DATA_BLOCK "DB_Gest_ES"
TITLE =
{ S7_language := '9(1) Angielski (Stany Zjednoczone)  11.01.2022  09:45:15' }
VERSION : 0.1


  STRUCT
   CMD : STRUCT
    StartVentilazione_Zona1 : BOOL ;	//Zona 1 +31FAN01
    StartVentilazione_Zona2 : BOOL ;	//Zona 2 +71FAN01
    SPARE_CMD0_02 : BOOL ;
    SPARE_CMD0_03 : BOOL ;
    StopVentilazione_Zona1 : BOOL ;
    StopVentilazione_Zona2 : BOOL ;
    VentilazioneRid_Zona1 : BOOL ;	//Ventilazione Ridotta Zona1
    VentilazioneRid_Zona2 : BOOL ;	//Ventilazione Ridotta Zona2
    Start_Riscarldo_Forno1 : BOOL ;
    Start_Riscarldo_Forno2 : BOOL ;
    AssenzaScoccheCabina : BOOL ;	//Assenza scocche cabina smalto
    SPARE_CMD1_03 : BOOL ;
    Stop_Riscarldo_Forno1 : BOOL ;
    Stop_Riscarldo_Forno2 : BOOL ;
    SPARE_CMD1_06 : BOOL ;
    SPARE_CMD1_07 : BOOL ;
    SPARE_CMD2_00 : BOOL ;
    SPARE_CMD2_01 : BOOL ;
    Forno2_PE_In_CMD2_02 : BOOL ;	//Scocca in ingresso Forno 2
    SPARE_CMD2_03 : BOOL ;
    SPARE_CMD2_04 : BOOL ;
    SPARE_CMD2_05 : BOOL ;
    SPARE_CMD2_06 : BOOL ;
    SPARE_CMD2_07 : BOOL ;
    SPARE_CMD3_00 : BOOL ;
    SPARE_CMD3_01 : BOOL ;
    SPARE_CMD3_02 : BOOL ;
    SPARE_CMD3_03 : BOOL ;
    SPARE_CMD3_04 : BOOL ;
    SPARE_CMD3_05 : BOOL ;
    SPARE_CMD3_06 : BOOL ;
    SPARE_CMD3_07 : BOOL ;
   END_STRUCT ;
   STS : STRUCT
    SPARE_STS0_00 : BOOL ;
    SPARE_STS0_01 : BOOL ;
    SPARE_STS0_02 : BOOL ;
    SPARE_STS0_03 : BOOL ;
    SPARE_STS0_04 : BOOL ;
    SPARE_STS0_05 : BOOL ;
    SPARE_STS0_06 : BOOL ;
    SPARE_STS0_07 : BOOL ;
    SPARE_STS1_00 : BOOL ;
    SPARE_STS1_01 : BOOL ;
    SPARE_STS1_02 : BOOL ;
    SPARE_STS1_03 : BOOL ;
    SPARE_STS1_04 : BOOL ;
    SPARE_STS1_05 : BOOL ;
    SPARE_STS1_06 : BOOL ;
    SPARE_STS1_07 : BOOL ;
    SPARE_STS2_00 : BOOL ;
    SPARE_STS2_01 : BOOL ;
    SPARE_STS2_02 : BOOL ;
    SPARE_STS2_03 : BOOL ;
    SPARE_STS2_04 : BOOL ;
    SPARE_STS2_05 : BOOL ;
    SPARE_STS2_06 : BOOL ;
    SPARE_STS2_07 : BOOL ;
    SPARE_STS3_00 : BOOL ;
    SPARE_STS3_01 : BOOL ;
    SPARE_STS3_02 : BOOL ;
    SPARE_STS3_03 : BOOL ;
    SPARE_STS3_04 : BOOL ;
    SPARE_STS3_05 : BOOL ;
    SPARE_STS3_06 : BOOL ;
    SPARE_STS3_07 : BOOL ;
   END_STRUCT ;
   Cnt_9PU1 : INT ;
   Cnt_8PU1 : INT ;
   Cnt_9RC : INT ;
   Cnt_8RC : INT ;
   Soglie : ARRAY  [1 .. 20 ] OF INT ;
   SetPoint : ARRAY  [1 .. 20 ] OF INT ;
   SPARE : ARRAY  [1 .. 20 ] OF INT ;
   FLAG : STRUCT
    _000 : BOOL ;	//Abilita Gestione Risparmio Energetico
    _001 : BOOL ;	//Stop Raffreddamento Linea 1
    _002 : BOOL ;	//Stop Raffreddamento Linea 2
    _003 : BOOL ;	//Stop Riscaldamento Linea 1
    _004 : BOOL ;	//Stop Riscaldamento Linea 2
    _005 : BOOL ;	//Forno 2 spento da Calendario
    _006 : BOOL ;	//RESERVE
    _007 : BOOL ;	//RESERVE
    _008 : BOOL ;	//RESERVE
    _009 : BOOL ;	//RESERVE
    _010 : BOOL ;	//RESERVE
    _011 : BOOL ;	//START COOLING ZONE Linea 1
    _012 : BOOL ;	//START COOLING ZONE Linea 2
    _013 : BOOL ;	//Start Raffreddamento Linea 1
    _014 : BOOL ;	//Start Raffreddamento Linea 2
    _015 : BOOL ;	//RESERVE
    _016 : BOOL ;	//RESERVE
    _017 : BOOL ;	//RESERVE
    _018 : BOOL ;	//RESERVE
    _019 : BOOL ;	//RESERVE
    _020 : BOOL ;	//RESERVE
    _021 : BOOL ;	//Riduzione Frequenza Raffreddamento Linea 1
    _022 : BOOL ;	//Riduzione Frequenza Raffreddamento Linea 2
    _023 : BOOL ;	//RESERVE
    _024 : BOOL ;	//RESERVE
    _025 : BOOL ;	//RESERVE
    _026 : BOOL ;	//RESERVE
    _027 : BOOL ;	//RESERVE
    _028 : BOOL ;	//RESERVE
    _029 : BOOL ;	//RESERVE
    _030 : BOOL ;	//AUX CONSENSO ACCENZIONE PRIMER
    _031 : BOOL ;	//ONS COMANDO ACCENSIONE PRIMER
    _032 : BOOL ;	//CMD STOP PRIMER
    _033 : BOOL ;	//Comando Accensione Manuale
    _034 : BOOL ;	//RESERVE
    _035 : BOOL ;	//RESERVE
    _036 : BOOL ;	//RESERVE
    _037 : BOOL ;	//RESERVE
    _038 : BOOL ;	//RESERVE
    _039 : BOOL ;	//AUX CONSENSO ACCENZIONE FORNO 2
    _040 : BOOL ;	//AUX CONSENSO ACCENZIONE FORNO 1
    _041 : BOOL ;	//ONS COMANDO ACCENSIONE FORNO 2
    _042 : BOOL ;	//ONS COMANDO ACCENSIONE FORNO 1
    _043 : BOOL ;	//RESERVE
    _044 : BOOL ;	//RESERVE
    _045 : BOOL ;	//RESERVE
    _046 : BOOL ;	//RESERVE
    _047 : BOOL ;	//RESERVE
    _048 : BOOL ;	//RESERVE
    _049 : BOOL ;	//RESERVE
    _050 : BOOL ;	//Ons Comando OFF senza calendario
    _051 : BOOL ;	//RESERVE
    _052 : BOOL ;	//RESERVE
    _053 : BOOL ;	//RESERVE
    _054 : BOOL ;	//RESERVE
    _055 : BOOL ;	//RESERVE
    _056 : BOOL ;	//RESERVE
    _057 : BOOL ;	//RESERVE
    _058 : BOOL ;	//RESERVE
    _059 : BOOL ;	//RESERVE
    _060 : BOOL ;	//RESERVE
    _061 : BOOL ;	//RESERVE
    _062 : BOOL ;	//RESERVE
    _063 : BOOL ;	//RESERVE
    _064 : BOOL ;	//RESERVE
    _065 : BOOL ;	//RESERVE
    _066 : BOOL ;	//RESERVE
    _067 : BOOL ;	//RESERVE
    _068 : BOOL ;	//RESERVE
    _069 : BOOL ;	//Abilita Gestione Risparmio Energetico FLA
    _070 : BOOL ;	//Start 43FLA02
    _071 : BOOL ;	//Start 44FLA02
    _072 : BOOL ;	//Start 51FLA02
    _073 : BOOL ;	//Start 52FLA02
    _074 : BOOL ;	//RESERVE
    _075 : BOOL ;	//RESERVE
    _076 : BOOL ;	//RESERVE
    _077 : BOOL ;	//Estate
    _078 : BOOL ;	//Temperato
    _079 : BOOL ;	//Inverno
    _080 : BOOL ;	//Modalita 1 Estate
    _081 : BOOL ;	//Modalita 1 Inverno
    _082 : BOOL ;	//Stop gruppo 84PP31-M1
    _083 : BOOL ;	//RESERVE
    _084 : BOOL ;	//RESERVE
    _085 : BOOL ;	//RESERVE
    _086 : BOOL ;	//RESERVE
    _087 : BOOL ;	//RESERVE
    _088 : BOOL ;	//RESERVE
    _089 : BOOL ;	//RESERVE
    _090 : BOOL ;	//RESERVE
    _091 : BOOL ;	//RESERVE
    _092 : BOOL ;	//RESERVE
    _093 : BOOL ;	//RESERVE
    _094 : BOOL ;	//RESERVE
    _095 : BOOL ;	//RESERVE
    _096 : BOOL ;	//RESERVE
    _097 : BOOL ;	//RESERVE
    _098 : BOOL ;	//RESERVE
    _099 : BOOL ;	//RESERVE
    _100 : BOOL ;	//RESERVE
   END_STRUCT ;
   ONS : ARRAY  [1 .. 20 ] OF BOOL ;
   Tmr : STRUCT
    Delay_01 : INT ;	//TMR Delay
    ONS_Delay_01 : BOOL ;	//Ons TMR Delay
    EN_Delay_01 : BOOL ;	//En TMR Delay
    DN_Delay_01 : BOOL ;	//DN TMR Delay
    Delay_02 : INT ;	//TMR Delay
    ONS_Delay_02 : BOOL ;	//Ons TMR Delay
    EN_Delay_02 : BOOL ;	//En TMR Delay
    DN_Delay_02 : BOOL ;	//DN TMR Delay
    Delay_03 : INT ;	//TMR Delay
    ONS_Delay_03 : BOOL ;	//Ons TMR Delay
    EN_Delay_03 : BOOL ;	//En TMR Delay
    DN_Delay_03 : BOOL ;	//DN TMR Delay
    Delay_04 : INT ;	//TMR Delay
    ONS_Delay_04 : BOOL ;	//Ons TMR Delay
    EN_Delay_04 : BOOL ;	//En TMR Delay
    DN_Delay_04 : BOOL ;	//DN TMR Delay
    Delay_05 : INT ;	//TMR Delay
    ONS_Delay_05 : BOOL ;	//Ons TMR Delay
    EN_Delay_05 : BOOL ;	//En TMR Delay
    DN_Delay_05 : BOOL ;	//DN TMR Delay
    Delay_06 : INT ;	//TMR Delay
    ONS_Delay_06 : BOOL ;	//Ons TMR Delay
    EN_Delay_06 : BOOL ;	//En TMR Delay
    DN_Delay_06 : BOOL ;	//DN TMR Delay
    Delay_07 : INT ;	//TMR Delay
    ONS_Delay_07 : BOOL ;	//Ons TMR Delay
    EN_Delay_07 : BOOL ;	//En TMR Delay
    DN_Delay_07 : BOOL ;	//DN TMR Delay
    Delay_08 : INT ;	//TMR Delay
    ONS_Delay_08 : BOOL ;	//Ons TMR Delay
    EN_Delay_08 : BOOL ;	//En TMR Delay
    DN_Delay_08 : BOOL ;	//DN TMR Delay
    Delay_09 : INT ;	//TMR Delay
    ONS_Delay_09 : BOOL ;	//Ons TMR Delay
    EN_Delay_09 : BOOL ;	//En TMR Delay
    DN_Delay_09 : BOOL ;	//DN TMR Delay
    Delay_10 : INT ;	//TMR Delay
    ONS_Delay_10 : BOOL ;	//Ons TMR Delay
    EN_Delay_10 : BOOL ;	//En TMR Delay
    DN_Delay_10 : BOOL ;	//DN TMR Delay
   END_STRUCT ;
  END_STRUCT ;
BEGIN
   CMD.StartVentilazione_Zona1 := FALSE;
   CMD.StartVentilazione_Zona2 := FALSE;
   CMD.SPARE_CMD0_02 := FALSE;
   CMD.SPARE_CMD0_03 := FALSE;
   CMD.StopVentilazione_Zona1 := TRUE;
   CMD.StopVentilazione_Zona2 := TRUE;
   CMD.VentilazioneRid_Zona1 := TRUE;
   CMD.VentilazioneRid_Zona2 := TRUE;
   CMD.Start_Riscarldo_Forno1 := FALSE;
   CMD.Start_Riscarldo_Forno2 := FALSE;
   CMD.AssenzaScoccheCabina := FALSE;
   CMD.SPARE_CMD1_03 := FALSE;
   CMD.Stop_Riscarldo_Forno1 := TRUE;
   CMD.Stop_Riscarldo_Forno2 := TRUE;
   CMD.SPARE_CMD1_06 := FALSE;
   CMD.SPARE_CMD1_07 := FALSE;
   CMD.SPARE_CMD2_00 := FALSE;
   CMD.SPARE_CMD2_01 := FALSE;
   CMD.Forno2_PE_In_CMD2_02 := FALSE;
   CMD.SPARE_CMD2_03 := FALSE;
   CMD.SPARE_CMD2_04 := FALSE;
   CMD.SPARE_CMD2_05 := FALSE;
   CMD.SPARE_CMD2_06 := FALSE;
   CMD.SPARE_CMD2_07 := FALSE;
   CMD.SPARE_CMD3_00 := FALSE;
   CMD.SPARE_CMD3_01 := FALSE;
   CMD.SPARE_CMD3_02 := FALSE;
   CMD.SPARE_CMD3_03 := FALSE;
   CMD.SPARE_CMD3_04 := FALSE;
   CMD.SPARE_CMD3_05 := FALSE;
   CMD.SPARE_CMD3_06 := FALSE;
   CMD.SPARE_CMD3_07 := FALSE;
   STS.SPARE_STS0_00 := FALSE;
   STS.SPARE_STS0_01 := FALSE;
   STS.SPARE_STS0_02 := FALSE;
   STS.SPARE_STS0_03 := FALSE;
   STS.SPARE_STS0_04 := FALSE;
   STS.SPARE_STS0_05 := FALSE;
   STS.SPARE_STS0_06 := FALSE;
   STS.SPARE_STS0_07 := FALSE;
   STS.SPARE_STS1_00 := FALSE;
   STS.SPARE_STS1_01 := FALSE;
   STS.SPARE_STS1_02 := FALSE;
   STS.SPARE_STS1_03 := FALSE;
   STS.SPARE_STS1_04 := FALSE;
   STS.SPARE_STS1_05 := FALSE;
   STS.SPARE_STS1_06 := FALSE;
   STS.SPARE_STS1_07 := FALSE;
   STS.SPARE_STS2_00 := FALSE;
   STS.SPARE_STS2_01 := FALSE;
   STS.SPARE_STS2_02 := FALSE;
   STS.SPARE_STS2_03 := FALSE;
   STS.SPARE_STS2_04 := FALSE;
   STS.SPARE_STS2_05 := FALSE;
   STS.SPARE_STS2_06 := FALSE;
   STS.SPARE_STS2_07 := FALSE;
   STS.SPARE_STS3_00 := FALSE;
   STS.SPARE_STS3_01 := FALSE;
   STS.SPARE_STS3_02 := FALSE;
   STS.SPARE_STS3_03 := FALSE;
   STS.SPARE_STS3_04 := FALSE;
   STS.SPARE_STS3_05 := FALSE;
   STS.SPARE_STS3_06 := FALSE;
   STS.SPARE_STS3_07 := FALSE;
   Cnt_9PU1 := 0;
   Cnt_8PU1 := 0;
   Cnt_9RC := 0;
   Cnt_8RC := 0;
   Soglie[1] := 0;
   Soglie[2] := 0;
   Soglie[3] := 0;
   Soglie[4] := 0;
   Soglie[5] := 0;
   Soglie[6] := 0;
   Soglie[7] := 0;
   Soglie[8] := 0;
   Soglie[9] := 0;
   Soglie[10] := 0;
   Soglie[11] := 0;
   Soglie[12] := 0;
   Soglie[13] := 0;
   Soglie[14] := 0;
   Soglie[15] := 0;
   Soglie[16] := 0;
   Soglie[17] := 0;
   Soglie[18] := 0;
   Soglie[19] := 0;
   Soglie[20] := 0;
   SetPoint[1] := 1800;
   SetPoint[2] := 1800;
   SetPoint[3] := 0;
   SetPoint[4] := 1500;
   SetPoint[5] := 60;
   SetPoint[6] := 60;
   SetPoint[7] := 100;
   SetPoint[8] := 200;
   SetPoint[9] := 3600;
   SetPoint[10] := 0;
   SetPoint[11] := 0;
   SetPoint[12] := 0;
   SetPoint[13] := 0;
   SetPoint[14] := 0;
   SetPoint[15] := 0;
   SetPoint[16] := 0;
   SetPoint[17] := 0;
   SetPoint[18] := 0;
   SetPoint[19] := 0;
   SetPoint[20] := 0;
   SPARE[1] := 0;
   SPARE[2] := 0;
   SPARE[3] := 0;
   SPARE[4] := 0;
   SPARE[5] := 0;
   SPARE[6] := 0;
   SPARE[7] := 0;
   SPARE[8] := 0;
   SPARE[9] := 0;
   SPARE[10] := 0;
   SPARE[11] := 0;
   SPARE[12] := 0;
   SPARE[13] := 0;
   SPARE[14] := 0;
   SPARE[15] := 0;
   SPARE[16] := 0;
   SPARE[17] := 0;
   SPARE[18] := 0;
   SPARE[19] := 0;
   SPARE[20] := 0;
   FLAG._000 := TRUE;
   FLAG._001 := FALSE;
   FLAG._002 := FALSE;
   FLAG._003 := FALSE;
   FLAG._004 := FALSE;
   FLAG._005 := FALSE;
   FLAG._006 := FALSE;
   FLAG._007 := FALSE;
   FLAG._008 := FALSE;
   FLAG._009 := FALSE;
   FLAG._010 := FALSE;
   FLAG._011 := FALSE;
   FLAG._012 := FALSE;
   FLAG._013 := TRUE;
   FLAG._014 := TRUE;
   FLAG._015 := FALSE;
   FLAG._016 := FALSE;
   FLAG._017 := FALSE;
   FLAG._018 := FALSE;
   FLAG._019 := FALSE;
   FLAG._020 := FALSE;
   FLAG._021 := FALSE;
   FLAG._022 := FALSE;
   FLAG._023 := FALSE;
   FLAG._024 := FALSE;
   FLAG._025 := FALSE;
   FLAG._026 := FALSE;
   FLAG._027 := FALSE;
   FLAG._028 := FALSE;
   FLAG._029 := FALSE;
   FLAG._030 := TRUE;
   FLAG._031 := FALSE;
   FLAG._032 := FALSE;
   FLAG._033 := FALSE;
   FLAG._034 := FALSE;
   FLAG._035 := FALSE;
   FLAG._036 := FALSE;
   FLAG._037 := FALSE;
   FLAG._038 := FALSE;
   FLAG._039 := TRUE;
   FLAG._040 := TRUE;
   FLAG._041 := FALSE;
   FLAG._042 := FALSE;
   FLAG._043 := FALSE;
   FLAG._044 := FALSE;
   FLAG._045 := FALSE;
   FLAG._046 := FALSE;
   FLAG._047 := FALSE;
   FLAG._048 := FALSE;
   FLAG._049 := FALSE;
   FLAG._050 := FALSE;
   FLAG._051 := FALSE;
   FLAG._052 := FALSE;
   FLAG._053 := FALSE;
   FLAG._054 := FALSE;
   FLAG._055 := FALSE;
   FLAG._056 := FALSE;
   FLAG._057 := FALSE;
   FLAG._058 := FALSE;
   FLAG._059 := FALSE;
   FLAG._060 := FALSE;
   FLAG._061 := FALSE;
   FLAG._062 := FALSE;
   FLAG._063 := FALSE;
   FLAG._064 := FALSE;
   FLAG._065 := FALSE;
   FLAG._066 := FALSE;
   FLAG._067 := FALSE;
   FLAG._068 := FALSE;
   FLAG._069 := FALSE;
   FLAG._070 := FALSE;
   FLAG._071 := FALSE;
   FLAG._072 := FALSE;
   FLAG._073 := FALSE;
   FLAG._074 := FALSE;
   FLAG._075 := FALSE;
   FLAG._076 := FALSE;
   FLAG._077 := FALSE;
   FLAG._078 := FALSE;
   FLAG._079 := FALSE;
   FLAG._080 := FALSE;
   FLAG._081 := FALSE;
   FLAG._082 := FALSE;
   FLAG._083 := FALSE;
   FLAG._084 := FALSE;
   FLAG._085 := FALSE;
   FLAG._086 := FALSE;
   FLAG._087 := FALSE;
   FLAG._088 := FALSE;
   FLAG._089 := FALSE;
   FLAG._090 := FALSE;
   FLAG._091 := FALSE;
   FLAG._092 := FALSE;
   FLAG._093 := FALSE;
   FLAG._094 := FALSE;
   FLAG._095 := FALSE;
   FLAG._096 := FALSE;
   FLAG._097 := FALSE;
   FLAG._098 := FALSE;
   FLAG._099 := FALSE;
   FLAG._100 := FALSE;
   ONS[1] := FALSE;
   ONS[2] := FALSE;
   ONS[3] := FALSE;
   ONS[4] := FALSE;
   ONS[5] := FALSE;
   ONS[6] := FALSE;
   ONS[7] := FALSE;
   ONS[8] := FALSE;
   ONS[9] := FALSE;
   ONS[10] := FALSE;
   ONS[11] := FALSE;
   ONS[12] := FALSE;
   ONS[13] := FALSE;
   ONS[14] := FALSE;
   ONS[15] := FALSE;
   ONS[16] := FALSE;
   ONS[17] := FALSE;
   ONS[18] := FALSE;
   ONS[19] := FALSE;
   ONS[20] := FALSE;
   Tmr.Delay_01 := 0;
   Tmr.ONS_Delay_01 := FALSE;
   Tmr.EN_Delay_01 := FALSE;
   Tmr.DN_Delay_01 := FALSE;
   Tmr.Delay_02 := 0;
   Tmr.ONS_Delay_02 := FALSE;
   Tmr.EN_Delay_02 := FALSE;
   Tmr.DN_Delay_02 := FALSE;
   Tmr.Delay_03 := 0;
   Tmr.ONS_Delay_03 := FALSE;
   Tmr.EN_Delay_03 := FALSE;
   Tmr.DN_Delay_03 := FALSE;
   Tmr.Delay_04 := 0;
   Tmr.ONS_Delay_04 := FALSE;
   Tmr.EN_Delay_04 := FALSE;
   Tmr.DN_Delay_04 := FALSE;
   Tmr.Delay_05 := 0;
   Tmr.ONS_Delay_05 := FALSE;
   Tmr.EN_Delay_05 := FALSE;
   Tmr.DN_Delay_05 := FALSE;
   Tmr.Delay_06 := 0;
   Tmr.ONS_Delay_06 := FALSE;
   Tmr.EN_Delay_06 := FALSE;
   Tmr.DN_Delay_06 := FALSE;
   Tmr.Delay_07 := 0;
   Tmr.ONS_Delay_07 := FALSE;
   Tmr.EN_Delay_07 := FALSE;
   Tmr.DN_Delay_07 := FALSE;
   Tmr.Delay_08 := 0;
   Tmr.ONS_Delay_08 := FALSE;
   Tmr.EN_Delay_08 := FALSE;
   Tmr.DN_Delay_08 := FALSE;
   Tmr.Delay_09 := 0;
   Tmr.ONS_Delay_09 := FALSE;
   Tmr.EN_Delay_09 := FALSE;
   Tmr.DN_Delay_09 := FALSE;
   Tmr.Delay_10 := 0;
   Tmr.ONS_Delay_10 := FALSE;
   Tmr.EN_Delay_10 := FALSE;
   Tmr.DN_Delay_10 := FALSE;
END_DATA_BLOCK

